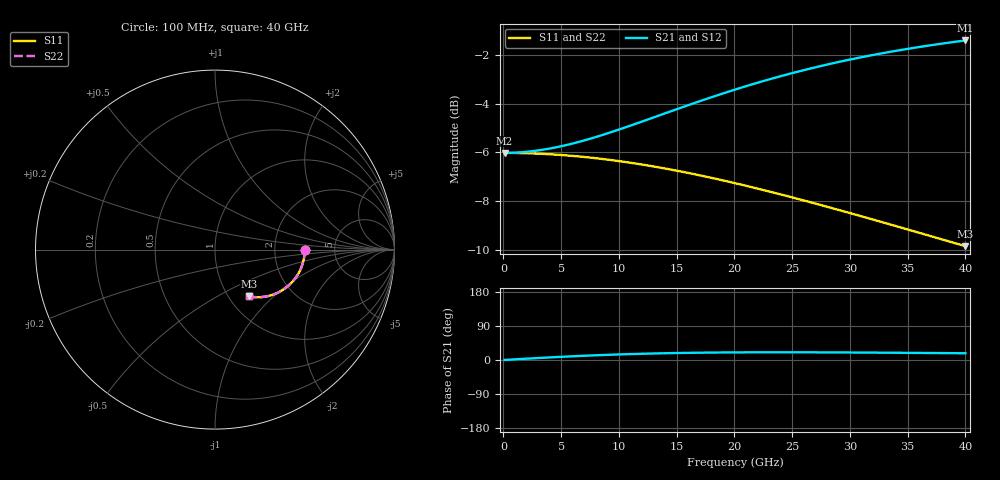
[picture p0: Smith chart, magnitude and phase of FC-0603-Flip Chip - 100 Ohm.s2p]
!Vishay Thin-Film
!FC Family
!Case Size 0603
!Assembly Style Flip Chip
!11/9/2015
!thinfilm@vishay.com
# GHz S MA R 50
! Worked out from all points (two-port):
!   101 points, 100 MHz to 40 GHz, reference 50 ohm
!   highest |S21| = -1.40 dB at 40 GHz (marker M1); lowest = -6.0 dB at 100 MHz (marker M2)
!   |S21| within 3 dB of the highest: 13.98 GHz to end of sweep
!   lowest |S11| = -9.9 dB at 40 GHz (marker M3), VSWR 1.95, Z = 61.8 - j35.9 ohm
!   |S11| at or under -10 dB: nowhere
!   |S22| runs from -9.9 to -6.0 dB; largest |S21 - S12| = 0
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0.1  0.5 -0.2  0.5 0.2  0.5 0.2  0.5 -0.2
1.696  0.4994 -3.0  0.5019 2.9  0.5019 2.9  0.4994 -3.0
3.292  0.4978 -5.7  0.5071 5.6  0.5071 5.6  0.4978 -5.7
4.888  0.4953 -8.5  0.5154 8.2  0.5154 8.2  0.4953 -8.5
6.883  0.4907 -11.9  0.5295 11.0  0.5295 11.0  0.4907 -11.9
8.479  0.4861 -14.6  0.5435 13.0  0.5435 13.0  0.4861 -14.6
10.474  0.4792 -17.9  0.5634 15.1  0.5634 15.1  0.4792 -17.9
12.07  0.4729 -20.4  0.5808 16.5  0.5808 16.5  0.4729 -20.4
13.666  0.4659 -22.9  0.5991 17.6  0.5991 17.6  0.4659 -22.9
15.262  0.4584 -25.4  0.6179 18.5  0.6179 18.5  0.4584 -25.4
16.858  0.4504 -27.8  0.637 19.2  0.637 19.2  0.4504 -27.8
18.454  0.442 -30.1  0.656 19.7  0.656 19.7  0.442 -30.1
20.05  0.4333 -32.3  0.6747 20.1  0.6747 20.1  0.4333 -32.3
21.646  0.4243 -34.4  0.693 20.3  0.693 20.3  0.4243 -34.4
23.242  0.4152 -36.5  0.7107 20.3  0.7107 20.3  0.4152 -36.5
24.838  0.406 -38.5  0.7278 20.3  0.7278 20.3  0.406 -38.5
26.833  0.3944 -40.9  0.748 20.2  0.748 20.2  0.3944 -40.9
28.429  0.3851 -42.8  0.7634 20.0  0.7634 20.0  0.3851 -42.8
30.025  0.3759 -44.5  0.778 19.8  0.778 19.8  0.3759 -44.5
33.616  0.3556 -48.2  0.8078 19.2  0.8078 19.2  0.3556 -48.2
36.808  0.3382 -51.2  0.8311 18.5  0.8311 18.5  0.3382 -51.2
40  0.3215 -54.0  0.8515 17.8  0.8515 17.8  0.3215 -54.0
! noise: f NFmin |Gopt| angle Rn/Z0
0.1  1.83e-07  1  -1.242e-17  2
4.489  1.707e-07  1  2.43e-15  1.865
8.878  1.422e-07  1  0  1.554
13.27  -3.857e-15  1  -1.207e-06  1.211
17.66  8.385e-08  1  4.153e-15  0.9162
22.05  6.31e-08  1  2.371e-14  0.6895
26.43  4.776e-08  1  -2.477e-14  0.5219
30.82  3.653e-08  1  -6.466e-15  0.3992
35.21  -4.822e-16  1  -1.915e-15  0.3089
40  4.333e-08  1  9.266e-15  0.2367
